(* Logix 5000 Rung export; software revision 16.03 *)

TYPE MCMEthernet :   // Stores the MVI56-MCM IP settings
STRUCT
   IP : INT[4];
   Netmask : INT[4];
   Gateway : INT[4];
END_STRUCT
END_TYPE

TYPE MCMEthernetType :   // Allows read/write Ethernet settings between the module and processor
STRUCT
   Read : BOOL;   // Enable Ethernet configuration transfer from module to processor
   Write : BOOL;   // Enable Ethernet configuration transfer from processor to module
   Config : MCMEthernet;
END_STRUCT
END_TYPE

TYPE MCMDateTime :   // Stores the date and time value
STRUCT
   Year : DINT;
   Month : DINT;
   Day : DINT;
   Hour : DINT;
   Minute : DINT;
   Seconds : DINT;
END_STRUCT
END_TYPE

TYPE MCMClockType :   // Allows read/write of clock value between the module and processor
STRUCT
   Read : BOOL;   // Reads current time from the module
   Write : BOOL;   // Writes current time from the module
   Config : MCMDateTime;   // Date and time configuration read or written between the module and processor
END_STRUCT
END_TYPE

ADD_ON_INSTRUCTION AOI56EMCM_Optional   (* revision 1.2, vendor ProSoft Technology Inc. *)
// MVI56E-MCM Optional Add-On Ethernet/Clock.
// Revision note:
// v1.2 - Updated name and description for standardization. No feature changes.
VAR_IN_OUT
   MVI56MCMEthernet : MCMEthernetType; {required}   // MVI56E-MCM Rev2 Ethernet Settings
   MVI56MCMClock : MCMClockType; {required}   // MVI56E-MCM Rev2 Clock Settings
   ReadEthernetMSG : MESSAGE; {required}   // Read Ethernet Settings Message
   WriteEthernetMSG : MESSAGE; {required}   // Write Ethernet Settings Message
   ReadClockMSG : MESSAGE; {required}   // Read Clock Settings Message
   WriteClockMSG : MESSAGE; {required}   // Write Clock Settings Message
END_VAR

ROUTINE Logic   (* ladder *)
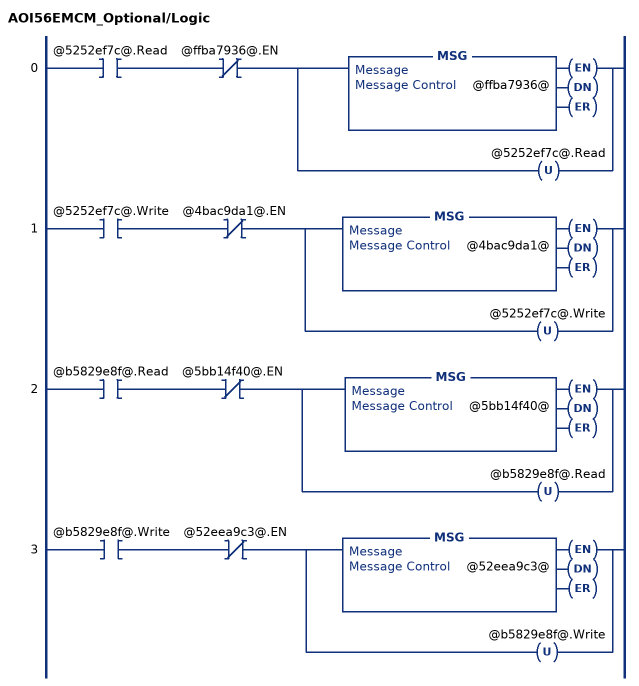
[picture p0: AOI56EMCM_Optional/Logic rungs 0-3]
   0: XIC(@5252ef7c@.Read)XIO(@ffba7936@.EN)[MSG(@ffba7936@) ,OTU(@5252ef7c@.Read) ];
   1: XIC(@5252ef7c@.Write)XIO(@4bac9da1@.EN)[MSG(@4bac9da1@) ,OTU(@5252ef7c@.Write) ];
   2: XIC(@b5829e8f@.Read)XIO(@5bb14f40@.EN)[MSG(@5bb14f40@) ,OTU(@b5829e8f@.Read) ];
   3: XIC(@b5829e8f@.Write)XIO(@52eea9c3@.EN)[MSG(@52eea9c3@) ,OTU(@b5829e8f@.Write) ];
END_ROUTINE
END_ADD_ON_INSTRUCTION

VAR_GLOBAL   (* controller tags *)
   WriteClockMSG : MESSAGE;
        MessageParameters(MessageType := CIP Generic, RequestedLength := 24, ConnectedFlag := 2, ConnectionPath := MCM, ServiceCode := 16#0010, ObjectType := 16#0004, TargetObject := 8, AttributeNumber := 16#0020, LocalElement := MVI56EMCMClock.Config)
   WriteEthernetMSG : MESSAGE;
        MessageParameters(MessageType := CIP Generic, RequestedLength := 24, ConnectedFlag := 2, ConnectionPath := MCM, ServiceCode := 16#0010, ObjectType := 16#0004, TargetObject := 8, LocalElement := MVI56EMCMEthernet.Config)
   AOI56EMCM_Optional : AOI56EMCM_Optional;
   MVI56EMCMEthernet : MCMEthernetType;
   ReadClockMSG : MESSAGE;
        MessageParameters(MessageType := CIP Generic, ConnectedFlag := 2, ConnectionPath := MCM, ServiceCode := 16#000e, ObjectType := 16#0004, TargetObject := 8, AttributeNumber := 16#0020, DestinationTag := MVI56EMCMClock.Config)
   MVI56EMCMClock : MCMClockType;
   ReadEthernetMSG : MESSAGE;
        MessageParameters(MessageType := CIP Generic, ConnectedFlag := 2, ConnectionPath := MCM, ServiceCode := 16#000e, ObjectType := 16#0004, TargetObject := 8, DestinationTag := MVI56EMCMEthernet.Config)
END_VAR

PROGRAM MainProgram

ROUTINE MainRoutine   (* ladder *)
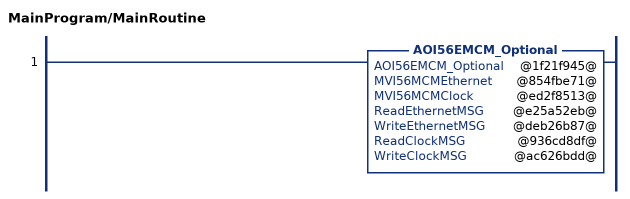
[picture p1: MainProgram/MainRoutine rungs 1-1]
   1: AOI56EMCM_Optional(@1f21f945@,@854fbe71@,@ed2f8513@,@e25a52eb@,@deb26b87@,@936cd8df@,@ac626bdd@);
END_ROUTINE
END_PROGRAM
